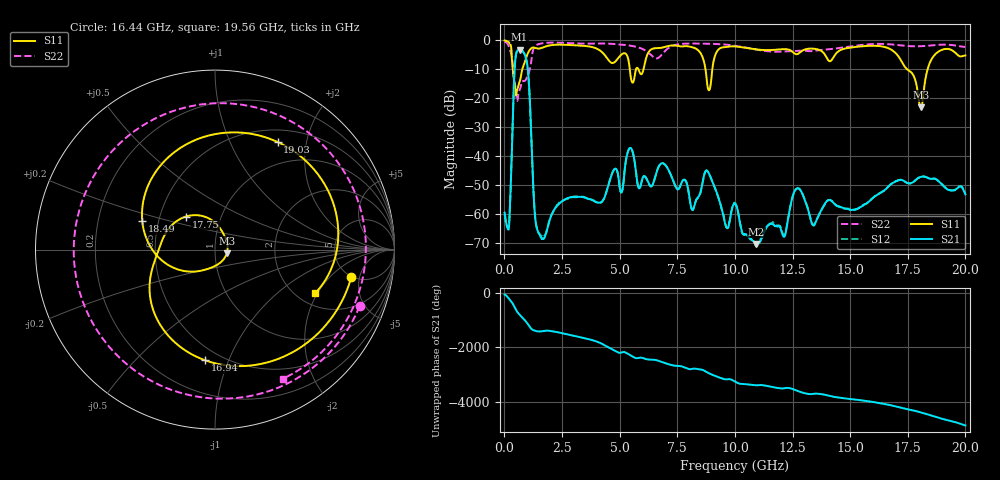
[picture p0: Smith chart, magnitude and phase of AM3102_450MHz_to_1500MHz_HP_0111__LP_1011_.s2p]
!Agilent Technologies,E8364B,MY43040894,A.07.50.67
!Agilent E8364B: A.07.50.67
!Date: Thursday, January 11, 2018 05:53:56
!Correction: S11(Full 2 Port(1,2))
!S21(Full 2 Port(1,2))
!S12(Full 2 Port(1,2))
!S22(Full 2 Port(1,2))
!S2P File: Measurements: S11, S21, S12, S22:
# Hz S  dB  R 50
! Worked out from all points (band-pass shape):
!   1601 points, 10 MHz to 20 GHz, reference 50 ohm
!   highest |S21| = -3.26 dB at 659.7 MHz (marker M1); lowest = -70.4 dB at 10.93 GHz (marker M2)
!   |S21| within 3 dB of the highest: 479.6 MHz to 936.6 MHz (456.9 MHz wide, 64.5 % of centre)
!   lowest |S11| = -23.2 dB at 18.06 GHz (marker M3), VSWR 1.15, Z = 57 - j2.41 ohm
!   |S11| at or under -10 dB: 365.3 MHz to 778.7 MHz (413.4 MHz wide, 72.3 % of centre); 8.724 GHz to 9.021 GHz (296.5 MHz wide, 3.34 % of centre); 17.47 GHz to 18.36 GHz (895.4 MHz wide, 5 % of centre)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
!   |S22| runs from -20.9 to -0.5 dB; largest |S21 - S12| = 0.0022
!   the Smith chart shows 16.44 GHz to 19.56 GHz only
!   S11 on the Smith chart (normalised r, x): 16.44 GHz: 4.91, -3.78; 16.94 GHz: 0.41, -0.83; 17.75 GHz: 0.68, +0.27; 18.49 GHz: 0.41, +0.16; 19.03 GHz: 0.66, +1.53; 19.56 GHz: 2.50, -1.91
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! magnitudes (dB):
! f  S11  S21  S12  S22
! 10 MHz  -0.1  -59.6  -60.3  -0.5
! 197.4 MHz  -0.7  -64.4  -63.8  -2.3
! 459.8 MHz  -16.3  -8.0  -8.0  -15.1
! 659.7 MHz  -14.4  -3.3  -3.3  -17.2
! 997 MHz  -4.9  -8.7  -8.7  -12.7
! 1.472 GHz  -2.9  -66.3  -66.3  -1.4
! 3.346 GHz  -1.9  -54.1  -54.0  -1.2
! 6.682 GHz  -2.7  -43.9  -43.9  -6.1
! 8.881 GHz  -17.3  -46.1  -46.2  -1.2
! 10.01 GHz  -2.1  -56.4  -56.2  -1.9
! 10.93 GHz  -3.1  -70.4  -71.0  -3.2
! 12.7 GHz  -4.8  -51.2  -51.1  -3.6
! 13.34 GHz  -2.9  -63.3  -63.2  -3.7
! 16.44 GHz  -2.2  -52.1  -52.1  -1.3
! 16.68 GHz  -2.8  -50.4  -50.4  -1.4
! 16.94 GHz  -4.2  -48.9  -48.9  -1.5
! 17.75 GHz  -12.2  -48.9  -48.9  -2.1
! 18.06 GHz  -23.2  -47.2  -47.2  -2.0
! 18.49 GHz  -7.2  -47.9  -47.9  -1.8
! 19.03 GHz  -3.2  -50.2  -50.1  -1.5
! 19.56 GHz  -4.3  -51.7  -51.6  -1.8
! 20 GHz  -5.2  -53.2  -53.0  -2.3
